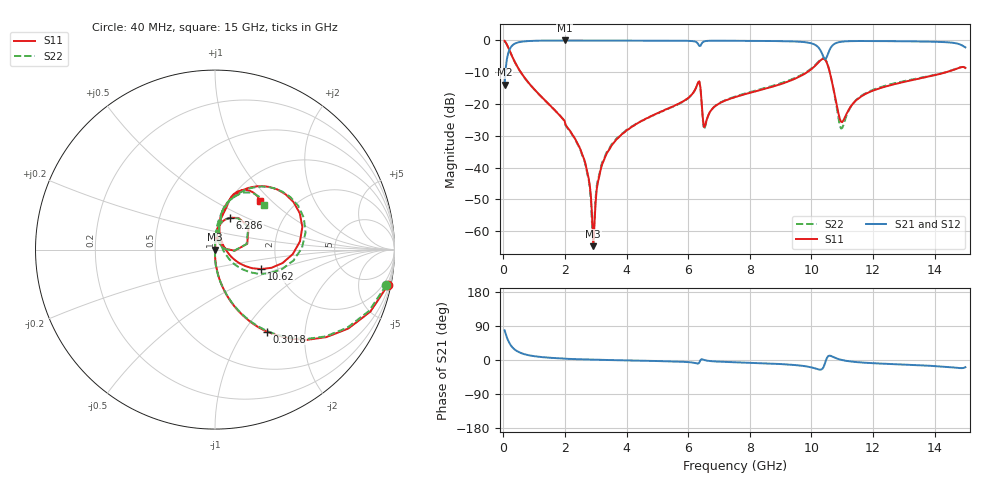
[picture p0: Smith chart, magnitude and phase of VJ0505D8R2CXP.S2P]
! VJ0505D8R2CXP
! MLCC placed on 25 mil thick microstrip substrate in series configuraton.
! DATE 06/29/2018  07:57
! CORRECTED  DATA
# GHz  S  MA  R  50.00
!  FREQ  S11M  S11A  S21M  S21A  S12M  S12A  S22M  S22A
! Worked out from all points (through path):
!   401 points, 40 MHz to 15 GHz, reference 50 ohm
!   highest |S21| = 0.00 dB at 1.985 GHz (marker M1); lowest = -13.9 dB at 40 MHz (marker M2)
!   group delay of S21, straight-line fit = 5.64 ps
!   lowest |S11| = -64.7 dB at 2.92 GHz (marker M3), VSWR 1.00, Z = 50.1 - j0.0256 ohm
!   |S11| at or under -10 dB: 566.3 MHz to 9.861 GHz (9.294 GHz wide, 178 % of centre); 10.6 GHz to 14.37 GHz (3.775 GHz wide, 30.2 % of centre)
!   |S22| runs from -64.4 to -0.2 dB; largest |S21 - S12| = 0.0017
!   S11 on the Smith chart (normalised r, x): 40 MHz: 0.84, -9.73; 301.8 MHz: 0.99, -1.28; 6.286 GHz: 1.11, +0.41; 10.62 GHz: 1.64, -0.39; 15 GHz: 1.36, +0.86
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0.04  0.9827 -11.7  0.2024 78.3  0.2026 78.3  0.9751 -11.6
0.3018  0.5399 -57.8  0.8448 32.7  0.8453 32.7  0.5353 -57.6
0.7132  0.2507 -76.3  0.971 14.7  0.9716 14.7  0.2488 -76.1
1.9848  0.05458 -88.6  1 3.7  1 3.7  0.05487 -90.0
2.5458  0.01681 -89.3  0.9987 1.7  0.9993 1.8  0.01642 -91.1
2.7328  0.008165 -88.4  0.9984 1.3  0.9994 1.3  0.007674 -94.4
2.9198  0.0005825 -26.0  0.9982 0.9  0.9991 0.9  0.0006003 160.8
3.1068  0.007088 83.1  0.9983 0.5  0.9985 0.5  0.007536 93.2
3.4434  0.01944 85.4  0.998 -0.1  0.9982 -0.1  0.02007 90.7
5.0516  0.07354 85.7  0.9953 -2.8  0.9956 -2.8  0.07285 87.7
6.2858  0.1969 64.4  0.9274 -9.3  0.9281 -9.3  0.1948 65.0
6.3606  0.2277 34.5  0.8193 -7.0  0.8201 -7.0  0.2241 34.2
6.5476  0.04537 56.6  0.9752 -0.6  0.9755 -0.6  0.04364 60.1
6.8842  0.09343 83.3  0.9914 -3.8  0.992 -3.8  0.09376 85.4
7.52  0.1286 82.9  0.9894 -5.9  0.9903 -5.9  0.1312 84.7
10.0258  0.3622 65.4  0.8933 -20.0  0.8948 -20.0  0.3724 63.2
10.3998  0.514 23.2  0.5425 -17.8  0.5429 -17.8  0.5255 19.6
10.6242  0.2792 -22.9  0.7624 11.0  0.763 11.0  0.2809 -28.9
10.9982  0.05195 30.4  0.9587 -0.1  0.9595 -0.1  0.04184 32.8
11.4844  0.1179 78.2  0.9803 -5.6  0.9807 -5.7  0.1197 79.1
12.5316  0.1958 77.6  0.9754 -10.4  0.9765 -10.5  0.202 79.3
15  0.3698 47.2  0.7793 -19.0  0.7801 -19.0  0.3703 42.4
